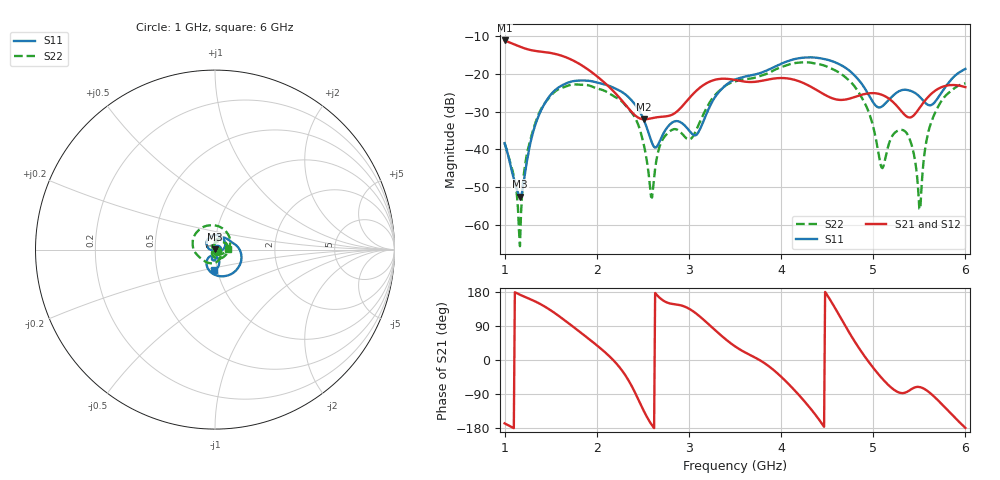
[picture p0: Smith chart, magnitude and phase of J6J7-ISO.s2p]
!Agilent Technologies,E8364B,MY43040528,A.07.50.67
!Agilent E8364B: A.07.50.67
!Date: Sunday, March 01, 2026 17:00:17
!Correction: S11(Full 2 Port(1,2))
!S21(Full 2 Port(1,2))
!S12(Full 2 Port(1,2))
!S22(Full 2 Port(1,2))
!S2P File: Measurements: S11, S21, S12, S22:
# Hz S  dB  R 50
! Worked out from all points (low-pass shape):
!   451 points, 1 GHz to 6 GHz, reference 50 ohm
!   highest |S21| = -11.18 dB at 1 GHz (marker M1); lowest = -32.0 dB at 2.511 GHz (marker M2)
!   |S21| within 3 dB of the highest: start of sweep to 1.41 GHz
!   lowest |S11| = -52.5 dB at 1.167 GHz (marker M3), VSWR 1.00, Z = 49.9 + j0.224 ohm
!   |S11| at or under -10 dB: start of sweep to end of sweep
!   |S22| runs from -65.6 to -16.9 dB; largest |S21 - S12| = 0.0011
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1e9  -38.32 25.1  -11.18 -167.2  -11.22 -167.2  -38.35 -32.5
1.166667e9  -52.47 109.4  -12.82 172.3  -12.85 172.3  -65.58 -151.8
1.244444e9  -42.76 -176.5  -13.48 164.0  -13.52 164.0  -40.64 158.5
1.377778e9  -30.62 178.0  -14.09 149.0  -14.12 149.1  -30.20 123.8
1.844444e9  -21.78 82.2  -17.88 68.8  -17.90 68.9  -22.89 -1.5
2.288889e9  -25.06 14.3  -27.54 -32.7  -27.56 -32.7  -27.71 -97.0
2.511111e9  -32.21 -14.5  -32.03 -134.8  -32.07 -134.7  -38.85 -160.4
2.588889e9  -37.57 -3.9  -31.78 -168.3  -31.82 -168.3  -52.53 115.0
2.666667e9  -38.70 39.8  -31.45 167.9  -31.48 167.9  -40.54 -0.4
2.844444e9  -32.59 47.3  -30.45 147.1  -30.48 147.1  -34.62 -51.9
3.088889e9  -35.96 72.3  -24.29 120.6  -24.33 120.7  -34.37 -30.7
3.5e9  -21.52 52.6  -21.62 36.1  -21.66 36.1  -22.03 -105.6
4.344444e9  -15.67 -51.3  -23.71 -135.7  -23.75 -135.6  -17.15 103.5
4.822222e9  -21.07 -122.4  -25.94 39.9  -25.98 40.0  -24.17 -11.6
4.966667e9  -26.25 -127.2  -25.13 -10.1  -25.16 -10.1  -31.21 -58.3
5.088889e9  -28.73 -98.3  -25.51 -46.7  -25.55 -46.7  -44.73 -160.3
5.166667e9  -26.94 -85.4  -26.51 -66.6  -26.54 -66.6  -38.80 101.4
5.366667e9  -24.27 -99.3  -31.35 -84.1  -31.39 -84.1  -35.82 26.8
5.511111e9  -26.25 -108.3  -28.75 -71.8  -28.78 -71.8  -55.78 86.6
5.577778e9  -27.96 -101.5  -26.61 -79.8  -26.65 -79.8  -37.65 121.4
5.655556e9  -27.83 -82.5  -24.77 -95.4  -24.81 -95.4  -31.14 102.9
6e9  -18.70 -92.0  -23.53 -179.2  -23.57 -179.2  -22.52 4.2
